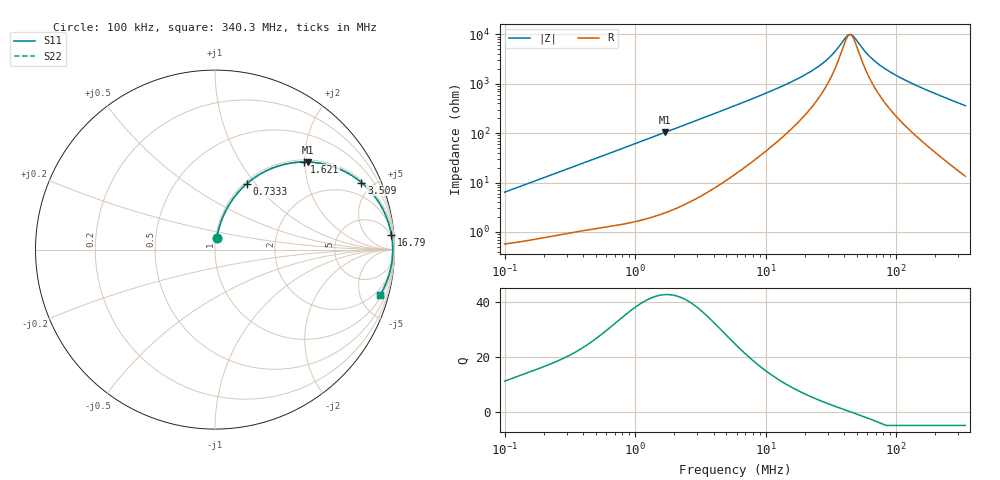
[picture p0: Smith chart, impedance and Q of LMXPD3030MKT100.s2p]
! LMXPD3030MKT100  S-PARAMETER MODEL  ( General Type )
! Model Generated by TAIYO YUDEN Corporation (https://www.yuden.co.jp/en/)
! Version 1.0
! TAIYO YUDEN Control No. 191023NI43SB-FBB
! Copyright(c) 2019 TAIYO YUDEN CO.,LTD. All Rights Reserved.
! Product Description (link to TY-COMPAS)
! https://ds.yuden.co.jp/TYCOMPAS/or/detail?pn=LMXPD3030MKT100M&u=M
! Products Name : Inductors
! Characteristics :
!  Inductance : 10 uH , SRF(min) : 32 MHz , DC Resistance(max) : 0.564 Ohm
!  Rated Current : Saturation :800 mA , Temp Rise : 550 mA (40 degC)
!  Case Size : 3.0 x 3.0 / 0.118 x 0.118 [mm/inch] , Thickness : 1.2 / 0.047 [mm/inch]
!  (Conditions: Temperature = 25 degC , DC Bias Current/Voltage = 0A / 0V)
! External Node Assignments :
!  1  o---GGG---o  2
! GND o---------o GND
! Frequency Range : 0.1MHz  -  340.31115MHz  [ 402 STEP ]
# MHz S RI R 50
! Freq[MHz].  S11 Real  S11 Imag  S21 Real  S21 Imag  S12 Real  S12 Imag  S22 Real  S22 Imag
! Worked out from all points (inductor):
!   401 points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, 100 kHz to 340.3 MHz, reference 50 ohm
!   read as one part in series: L = 10.1 uH near 104.2 kHz
!   highest Q = 42.6 at 1.688 MHz (marker M1), where L = 9.75 uH
!   self-resonance near 43.66 MHz
!   S11 on the Smith chart (normalised r, x): 100 kHz: 1.01, +0.13; 733.3 kHz: 1.03, +0.90; 1.621 MHz: 1.05, +1.99; 3.509 MHz: 1.12, +4.31; 16.79 MHz: 4, +24; 340.3 MHz: 1.27, -7.20
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0.1  0.00967 0.0627  0.9903 -0.0627  0.9903 -0.0627  0.00967 0.0627
0.207907  0.0242 0.1267  0.9758 -0.1267  0.9758 -0.1267  0.0242 0.1267
0.390471  0.0642 0.2244  0.9358 -0.2244  0.9358 -0.2244  0.0642 0.2244
0.733347  0.1766 0.3665  0.8234 -0.3665  0.8234 -0.3665  0.1766 0.3665
1.524679  0.467 0.4872  0.533 -0.4872  0.533 -0.4872  0.467 0.4872
1.620569  0.4967 0.4884  0.5033 -0.4884  0.5033 -0.4884  0.4967 0.4884
1.687823  0.5165 0.4881  0.4835 -0.4881  0.4835 -0.4881  0.5165 0.4881
2.336695  0.6685 0.4588  0.3315 -0.4588  0.3315 -0.4588  0.6685 0.4588
3.509101  0.8161 0.3734  0.1839 -0.3734  0.1839 -0.3734  0.8161 0.3734
5.953437  0.9231 0.2466  0.0769 -0.2466  0.0769 -0.2466  0.9231 0.2466
16.79121  0.9832 0.0814  0.0168 -0.0814  0.0168 -0.0814  0.9832 0.0814
22.77862  0.9873 0.0518  0.0127 -0.0518  0.0127 -0.0518  0.9873 0.0518
30.2791  0.9892 0.0284  0.0108 -0.0284  0.0108 -0.0284  0.9892 0.0284
34.91008  0.9898 0.0176  0.0102 -0.0176  0.0102 -0.0176  0.9898 0.0176
41.07602  0.99 0.00571  0.00995 -0.00571  0.00995 -0.00571  0.99 0.00571
44.5561  0.9901 -0.000177  0.00991 0.000177  0.00991 0.000177  0.9901 -0.000177
47.35831  0.9901 -0.00459  0.00993 0.00459  0.00993 0.00459  0.9901 -0.00459
56.86741  0.9898 -0.018  0.0102 0.018  0.0102 0.018  0.9898 -0.018
65.56488  0.9893 -0.0288  0.0107 0.0288  0.0107 0.0288  0.9893 -0.0288
88.94399  0.9871 -0.0541  0.0129 0.0541  0.0129 0.0541  0.9871 -0.0541
153.9991  0.9769 -0.1132  0.0231 0.1132  0.0231 0.1132  0.9769 -0.1132
340.3111  0.9204 -0.2527  0.0796 0.2527  0.0796 0.2527  0.9204 -0.2527
